(* Sampled values publisher *)
{attribute 'no_assign'}
FUNCTION_BLOCK FB_IED_MUnn_MSVCB02SvPublisher IMPLEMENTS I_GseLinkStatusEventSink
VAR_INPUT
	fbAdapter: FB_GseAdapterClass := (ipLinkStatus:=THIS^); (* GSE network adapter *)
	fbApdu1: FB_SVTXAPDU_IED_MUnn_LLN0_MSVCB02; (* SV publisher APDU *)
	(*
	fbApdu2: FB_SVTXAPDU_...
	...
	fbApduN: FB_SVTXAPDU_...
	*)
END_VAR
VAR
	eLinkStatus: E_GseLinkStatus; (* Network adapter link status *)
	bSuccess: BOOL;
	ipError: I_ServiceErrorClass;
	bStart: BOOL := TRUE; (* Rising edge starts publishing of SV data *)
	bStop: BOOL; (* Rising edge stops publishing of SV data *)
	bUpdate: BOOL := TRUE; (* Enable/disable cyclic update of published SV data. Default: TRUE (enabled) *)
	bUpdateOnce: BOOL; (* Rising edge updates published SV data only once *)
	
	bSynch: BOOL := TRUE; (* Rising edge at this input resets the sample counter to 0 *)
	nSynch: UDINT; (* Increments every time sampling is synchronized *)
	nSmpCnt: UINT; (* Sample counter *)
	eSmpSynch: E_GseSvSmpSynch := E_GseSvSmpSynch.Local; (* Synchronization type: 0..2 *)
	tRefrTm: T_UtcTime; (* Sample refresh time stamp (optional) *)
	qMeasure: ST_AcsiQuality := (Derived:=TRUE); (* SV quality bits *)
	bSimulation: BOOL := TRUE; (* Enable/disable SV test signal function generator. Default: TRUE (enabled) *)
	
	fbGenerator1: FB_GseSvPhsMeasGeneratorClass := (
		nOversampleFactor:=cOversampleFactor_IED_MUnn_LLN0_MSVCB02_Asdu1, (* Sets oversampling factor. Default: 1 (no oversampling) *)
		AmpA:=(fFrequency:=50.0, fAmplitude:=100, fPhi:=0),
		AmpB:=(fFrequency:=50.0, fAmplitude:=100, fPhi:=-120),
		AmpC:=(fFrequency:=50.0, fAmplitude:=100, fPhi:=-240),
		VolA:=(fFrequency:=50.0, fAmplitude:=230 * SQRT(2), fPhi:=0),
		VolB:=(fFrequency:=50.0, fAmplitude:=230 * SQRT(2), fPhi:=-120),
		VolC:=(fFrequency:=50.0, fAmplitude:=230 * SQRT(2), fPhi:=-240)); (* SV test signal function generator for PhsMeas1 dataset according to UCA 61850-9-2LE specification *)
END_VAR

bSuccess:= fbAdapter.Execute(ipError=>ipError); (* Execute network adapter *)

IF bStart THEN (* Start publishing of SV data *)
	bStart:= FALSE;
	fbGenerator1.Config(); (* Configure SV test signal function generator *)
	bSuccess:= fbIED.IEDMUnn.LLN0.MSVCB02.Publisher.Start(ipAdapter:=fbAdapter, ipApdu:=fbApdu1, ipError=>ipError);
ELSIF bStop THEN (* Stop publishing of SV data *)
	bStop:= FALSE;
	bSuccess:= fbIED.IEDMUnn.LLN0.MSVCB02.Publisher.Stop(ipError=>ipError);
ELSIF bUpdate OR_ELSE bUpdateOnce THEN (* Update published SV data *)
	bUpdateOnce:= FALSE;
	SvSimulation(); (* Create test signal SV data *)
	bSuccess:= fbIED.IEDMUnn.LLN0.MSVCB02.Publisher.Update(ipError=>ipError);
ELSE (* Execute publisher SvCB's *)
	bSuccess:= fbIED.IEDMUnn.LLN0.MSVCB02.Publisher.Execute(ipError=>ipError);
END_IF

{attribute 'analysis' := '-33'}
(* This method is called every time the network adapter link status changes *)
METHOD FINAL OnLinkStatusChange
VAR_INPUT
	ipAdapter: I_GseAdapterClass; (* Interface pointer of the network adapter reporting link status change *)
	eStatus: E_GseLinkStatus; (* New (changed) link status *)
END_VAR
VAR
END_VAR
eLinkStatus:= eStatus;
END_METHOD

(* Create SV test data. The data will be sent the next time when the publisher's Update() method is called *)
METHOD PRIVATE SvSimulation
VAR
	index: UINT; (* Temp. variable *)
END_VAR
fbApdu1.bSimulation:= bSimulation; (* Example => Sets SV ethernet header simulation flag *)
qMeasure.Test:= bSimulation; (* Example => Sets "Quality.Test" bit to TRUE if simulation enabled *)
qMeasure.Validity1:= NOT qMeasure.Validity1; (* Example => Toggle some "Quality.Validity" bits *)

FOR index:=0 TO cOversampleFactor_IED_MUnn_LLN0_MSVCB02_Asdu1-1 BY 1 DO
	IF bSynch THEN
		bSynch:= FALSE;
		nSmpCnt:= 0; (* Example => Set sample counter to 0 *)
		fbGenerator1.Reset(); (* Reset SV test signal function generator *)
		nSynch:= nSynch + 1;
	ELSE
		nSmpCnt:= nSmpCnt + 1; (* Increment sample counter *)
	END_IF

	IF bSimulation THEN
		fbGenerator1.Call(); (* Call SV test signal function generator for new data *)
	END_IF

	fbApdu1.TxData.Asdu1.nSmpCnt[index]:= nSmpCnt; (* Set sample counter *)
	fbApdu1.TxData.Asdu1.eSmpSynch[index]:= eSmpSynch; (* Set synchronization type: 0..2 *)
	(* Hint: The time stamp will only be sent if "RefreshTime" parameter in the "OptFlds" of the SV publisher control block is set to TRUE *)
	fbApdu1.TxData.Asdu1.tRefrTm[index]:= tRefrTm; (* Set sample refresh time stamp (optional) *)

	(* Include the following to simulate IEC 61850 9-2LE values. This only works if the rest of the datamodel complies with the standard.*)
	fbApdu1.TxData.Asdu1.IED_MUnn_InnATCTR1_AmpSv_instMag_i[index]:= SEL(bSimulation, 0, TO_DINT(fbGenerator1.AmpA.fSignal));
	fbApdu1.TxData.Asdu1.IED_MUnn_InnATCTR1_AmpSv_q[index]:= qMeasure;
	fbApdu1.TxData.Asdu1.IED_MUnn_InnBTCTR2_AmpSv_instMag_i[index]:= SEL(bSimulation, 0, TO_DINT(fbGenerator1.AmpB.fSignal));
	fbApdu1.TxData.Asdu1.IED_MUnn_InnBTCTR2_AmpSv_q[index]:= qMeasure;
	fbApdu1.TxData.Asdu1.IED_MUnn_InnCTCTR3_AmpSv_instMag_i[index]:= SEL(bSimulation, 0, TO_DINT(fbGenerator1.AmpC.fSignal));
	fbApdu1.TxData.Asdu1.IED_MUnn_InnCTCTR3_AmpSv_q[index]:= qMeasure;
	fbApdu1.TxData.Asdu1.IED_MUnn_InnNTCTR4_AmpSv_instMag_i[index]:= SEL(bSimulation, 0, TO_DINT(fbGenerator1.AmpA.fSignal + fbGenerator1.AmpB.fSignal + fbGenerator1.AmpC.fSignal));
	fbApdu1.TxData.Asdu1.IED_MUnn_InnNTCTR4_AmpSv_q[index]:= qMeasure;
	fbApdu1.TxData.Asdu1.IED_MUnn_UnnATVTR1_VolSv_instMag_i[index]:= SEL(bSimulation, 0, TO_DINT(fbGenerator1.VolA.fSignal));
	fbApdu1.TxData.Asdu1.IED_MUnn_UnnATVTR1_VolSv_q[index]:= qMeasure;
	fbApdu1.TxData.Asdu1.IED_MUnn_UnnBTVTR2_VolSv_instMag_i[index]:= SEL(bSimulation, 0, TO_DINT(fbGenerator1.VolB.fSignal));
	fbApdu1.TxData.Asdu1.IED_MUnn_UnnBTVTR2_VolSv_q[index]:= qMeasure;
	fbApdu1.TxData.Asdu1.IED_MUnn_UnnCTVTR3_VolSv_instMag_i[index]:= SEL(bSimulation, 0, TO_DINT(fbGenerator1.VolC.fSignal));
	fbApdu1.TxData.Asdu1.IED_MUnn_UnnCTVTR3_VolSv_q[index]:= qMeasure;
	fbApdu1.TxData.Asdu1.IED_MUnn_UnnNTVTR4_VolSv_instMag_i[index]:= SEL(bSimulation, 0, TO_DINT(fbGenerator1.VolA.fSignal + fbGenerator1.VolB.fSignal + fbGenerator1.VolC.fSignal));
	fbApdu1.TxData.Asdu1.IED_MUnn_UnnNTVTR4_VolSv_q[index]:= qMeasure;
END_FOR
END_METHOD

END_FUNCTION_BLOCK
